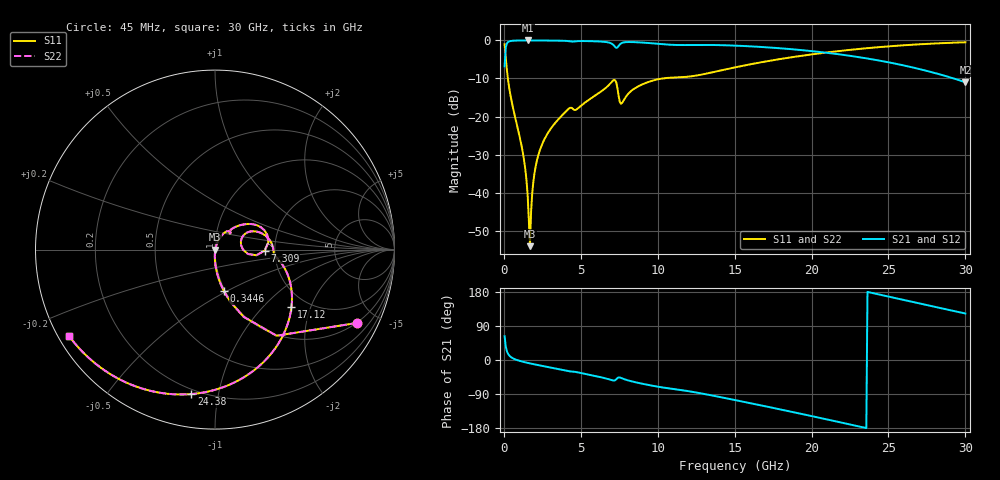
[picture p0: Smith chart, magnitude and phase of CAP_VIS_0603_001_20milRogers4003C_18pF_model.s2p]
! S-parameter model data by Modelithics Inc.  support@modelithics.com  813-866-6335  Tampa FL USA
! S-Parameter data specifications:
! Substrate: 20-mil Rogers 4003C, substrate thickness, H=0.508mm, Dielectric constant, Er=3.75
! PCB Mounting Pad Footprint: Pad width, PadW=0.90mm , Pad length, PadL=1.00mm , Pad gap, PadG (edge-to-edge)=1.00mm , Reference planes=3.0mm apart
! Created Wed Nov 18 13:27:01 2015
# hz S ma R 50
! 2 Port Network Data from SP1.SP block
! freq  magS11  angS11  magS21  angS21  magS12  angS12  magS22  angS22
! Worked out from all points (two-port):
!   401 points, 45 MHz to 30 GHz, reference 50 ohm
!   highest |S21| = -0.02 dB at 1.543 GHz (marker M1); lowest = -11.0 dB at 30 GHz (marker M2)
!   |S21| within 3 dB of the highest: 102.5 MHz to 20.47 GHz (20.37 GHz wide, 198 % of centre)
!   lowest |S11| = -54.1 dB at 1.693 GHz (marker M3), VSWR 1.00, Z = 50.2 + j0.0412 ohm
!   |S11| at or under -10 dB: 258.9 MHz to 10.32 GHz (10.06 GHz wide, 190 % of centre)
!   |S22| runs from -54.1 to -0.5 dB; largest |S21 - S12| = 0
!   S11 on the Smith chart (normalised r, x): 45 MHz: 0.98, -3.88; 344.6 MHz: 0.99, -0.49; 7.309 GHz: 1.77, -0.02; 17.12 GHz: 1.66, -1.48; 24.38 GHz: 0.17, -0.83; 30 GHz: 0.03, -0.27
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4.5e7  0.8903 -27.3  0.4553 62.7  0.4553 62.7  0.8903 -27.3
3.4455e8  0.2377 -77.9  0.9705 11.9  0.9705 11.9  0.2377 -77.9
1.2432e9  0.03232 -91.9  0.9978 -4.7  0.9978 -4.7  0.03232 -91.9
1.392975e9  0.02004 -91.4  0.998 -6.2  0.998 -6.2  0.02004 -91.4
1.54275e9  0.009277 -86.7  0.9981 -7.6  0.9981 -7.6  0.009277 -86.7
1.692525e9  0.001979 12.0  0.998 -9.0  0.998 -9.0  0.001979 12.0
1.767412e9  0.005634 60.8  0.9979 -9.6  0.9979 -9.6  0.005634 60.8
2.066962e9  0.02231 72.5  0.9975 -12.2  0.9975 -12.2  0.02231 72.5
2.591175e9  0.04831 70.7  0.9962 -16.4  0.9962 -16.4  0.04831 70.7
4.088925e9  0.1201 57.3  0.9836 -28.4  0.9836 -28.4  0.1201 57.3
5.062462e9  0.1414 51.4  0.9803 -34.8  0.9803 -34.8  0.1414 51.4
6.784875e9  0.2549 33.6  0.9403 -50.4  0.9403 -50.4  0.2549 33.6
7.309088e9  0.2772 -1.1  0.797 -50.7  0.797 -50.7  0.2772 -1.1
7.683525e9  0.1512 17.6  0.9282 -48.4  0.9282 -48.4  0.1512 17.6
8.582175e9  0.2394 25.3  0.9466 -59.0  0.9466 -59.0  0.2394 25.3
1.007992e10  0.3102 9.5  0.8997 -71.0  0.8997 -71.0  0.3102 9.5
1.50225e10  0.4421 -21.2  0.8539 -105.7  0.8539 -105.7  0.4421 -21.2
1.711935e10  0.5329 -36.9  0.8104 -123.2  0.8104 -123.2  0.5329 -36.9
2.003996e10  0.6558 -61.0  0.722 -148.3  0.722 -148.3  0.6558 -61.0
2.438344e10  0.8157 -99.3  0.5439 172.9  0.5439 172.9  0.8157 -99.3
2.505742e10  0.8364 -105.4  0.5128 166.8  0.5128 166.8  0.8364 -105.4
3e10  0.945 -149.5  0.2819 122.8  0.2819 122.8  0.945 -149.5
